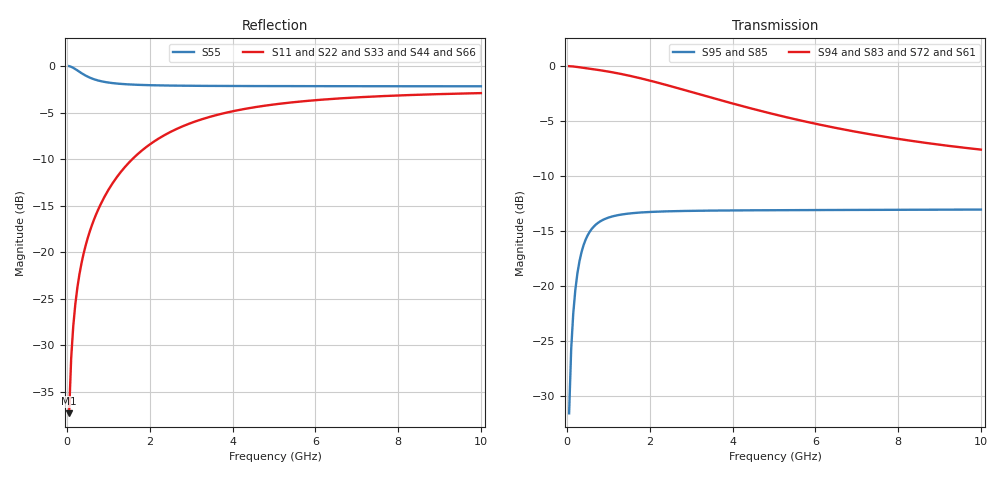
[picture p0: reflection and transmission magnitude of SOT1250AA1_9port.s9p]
! Created Wed Jan 16 16:31:29 2019
# ghz S ma R 50
! 9 Port Network Data from SP1.SP block
! freq  magS11  angS11  magS12  angS12  magS13  angS13  magS14  angS14
!  magS15  angS15  magS16  angS16  magS17  angS17  magS18  angS18
!  magS19  angS19
!  magS21  angS21  magS22  angS22  magS23  angS23
!  magS24  angS24  magS25  angS25  magS26  angS26  magS27  angS27
!  magS28  angS28  magS29  angS29
!  magS31  angS31  magS32  angS32
!  magS33  angS33  magS34  angS34  magS35  angS35  magS36  angS36
!  magS37  angS37  magS38  angS38  magS39  angS39
!  magS41  angS41
!  magS42  angS42  magS43  angS43  magS44  angS44  magS45  angS45
!  magS46  angS46  magS47  angS47  magS48  angS48  magS49  angS49
!  magS51  angS51  magS52  angS52  magS53  angS53  magS54  angS54
!  magS55  angS55  magS56  angS56  magS57  angS57  magS58  angS58
!  magS59  angS59
!  magS61  angS61  magS62  angS62  magS63  angS63
!  magS64  angS64  magS65  angS65  magS66  angS66  magS67  angS67
!  magS68  angS68  magS69  angS69
!  magS71  angS71  magS72  angS72
!  magS73  angS73  magS74  angS74  magS75  angS75  magS76  angS76
!  magS77  angS77  magS78  angS78  magS79  angS79
!  magS81  angS81
!  magS82  angS82  magS83  angS83  magS84  angS84  magS85  angS85
!  magS86  angS86  magS87  angS87  magS88  angS88  magS89  angS89
!  magS91  angS91  magS92  angS92  magS93  angS93  magS94  angS94
!  magS95  angS95  magS96  angS96  magS97  angS97  magS98  angS98
!  magS99  angS99
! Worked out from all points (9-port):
!   200 points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, 50 MHz to 10 GHz, reference 50 ohm
!   strongest paths, dB at 50 MHz, 2.55 GHz, 5.05 GHz, 7.55 GHz, 10 GHz:
!     S94: 0.0, -1.9, -4.4, -6.3, -7.6
!     S83: 0.0, -1.9, -4.4, -6.3, -7.6
!     S72: 0.0, -1.9, -4.4, -6.3, -7.6
!     S61: 0.0, -1.9, -4.4, -6.3, -7.6
!     S95: -31.5, -13.2, -13.1, -13.1, -13.0
!     S85: -31.5, -13.2, -13.1, -13.1, -13.0
!   lowest |S11| = -37.3 dB at 50 MHz (marker M1), VSWR 1.03, Z = 49.9 - j1.36 ohm
!   |S11| at or under -10 dB: start of sweep to 1.58 GHz
